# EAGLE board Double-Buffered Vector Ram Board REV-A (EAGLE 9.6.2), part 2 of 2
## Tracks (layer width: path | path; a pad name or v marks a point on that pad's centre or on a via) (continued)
VRAM_B_3 (continued)
  Top 0.508: 6E.13 212.81,13.34 214.08,12.06 216.45,12.06 217.72,13.34 7E.13 238.12,13.34 241.94,17.14 244.39,17.14 245.66,18.41 8E.12 9E.9
VRAM_B_4
  Top 0.508: 6E.14 208.88,15.88 210.15,14.61 216.45,14.61 217.72,15.88 7E.14 238.12,15.88 241.94,19.68 244.39,19.68 245.66,20.95 8E.13 9E.8
VRAM_B_5
  Top 0.508: 6E.15 208.88,18.41 210.15,17.14 216.45,17.14 217.72,18.41 7E.15 235.59,18.41 241.94,24.77 244.39,24.77 245.66,26.04 8E.15 9E.6
VRAM_B_6
  Top 0.508: 6E.16 208.88,20.95 210.15,19.68 216.45,19.68 217.72,20.95 7E.16 233.04,20.95 241.94,29.84 244.39,29.84 245.66,31.11 8E.17 9E.4
VRAM_B_7
  Top 0.508: 6E.17 208.88,23.5 210.15,22.23 216.45,22.23 217.72,23.5 7E.17 241.94,34.92 244.39,34.92 245.66,36.2 8E.19 9E.2
VRAM_B_8
  Top 0.508: 6C.9 205.19,61.59 206.46,62.87 208.83,62.87 210.1,61.59 7C.9 215.67,62 216.81,62 217.67,62.87 231.78,62.87 241.94,73.03 244.47,73.03 245.75,74.3 8C.18 9C.3
VRAM_B_9
  Top 0.508: 6C.10 205.19,59.05 206.46,60.33 208.83,60.33 210.1,59.05 7C.10 215.67,59.46 216.81,59.46 217.67,60.33 234.31,60.33 241.94,67.94 244.39,67.94 245.66,69.22 8C.16 9C.5
VRAM_B_10
  Top 0.508: 6C.11 205.19,56.52 206.46,57.78 208.83,57.78 210.1,56.52 7C.11 215.67,56.92 216.81,56.92 217.67,57.78 236.85,57.78 241.94,62.87 244.47,62.87 245.75,64.14 8C.14 9C.7
VRAM_B_11
  Top 0.381: 6C.13 207.72,53.77 208.83,52.67 229.08,52.67 230.19,53.77 7C.13
  Top 0.508: 7C.13 238.12,53.98 241.94,57.78 244.39,57.78 245.66,59.05 8C.12 9C.9
VRAM_B_12
  Top 0.508: 6C.14 208.88,56.52 210.15,55.24 216.45,55.24 217.72,56.52 7C.14 238.21,56.52 242.02,60.33 244.47,60.33 245.75,61.59 8C.13 9C.8
VRAM_B_13
  Top 0.508: 6C.15 208.88,59.05 210.15,57.78 216.45,57.78 217.72,59.05 7C.15 235.67,59.05 242.02,65.41 244.47,65.41 245.75,66.67 8C.15 9C.6
VRAM_B_14
  Top 0.508: 6C.16 208.88,61.59 210.15,60.33 216.45,60.33 217.72,61.59 7C.16 233.04,61.59 241.94,70.48 244.47,70.48 245.75,71.75 8C.17 9C.4
VRAM_B_15
  Top 0.508: 6C.17 208.88,64.14 210.15,62.87 216.45,62.87 217.72,64.14 7C.17 241.94,75.56 244.47,75.56 245.75,76.83 8C.19 9C.2
VRAMA0  (via drill 0.35)
  Top 0.381: v165.74,100.91 162.05,100.91 4B.11 161.68,101.28 v156.53,101.28 | v156.53,117.49 147.32,117.49 146.95,117.86 124.12,117.86 B1.49
  Bottom 0.381: v165.74,100.91 165.74,22.1 162.05,18.41 4E.11 | v156.53,101.28 v156.53,117.49
VRAMA1  (via drill 0.35)
  Top 0.381: v149.16,27.25 160.58,27.25 161.68,26.15 4E.14 | 4B.14 161.68,108.65 158,112.33 v148.79,112.33 145.11,108.65 119.7,108.65 119.7,116.38 121.17,117.86 B1.48
  Bottom 0.381: v149.16,27.25 149.16,73.29 148.43,74.03 148.43,111.96 v148.79,112.33
VRAMA2  (via drill 0.35)
  Top 0.381: v130.01,51.56 v175.31,51.56 | v130.01,120.43 124.12,120.43 B1.47 | v130.01,116.75 146.22,116.75 146.58,116.38 169.42,116.38 172,113.81 5B.5
  Bottom 0.381: v175.31,51.56 175.31,34.25 172.36,31.3 5E.5 | v130.01,120.43 v130.01,116.75 v130.01,51.56
VRAMA3  (via drill 0.35)
  Top 0.381: v183.78,42.72 176.05,42.72 172.36,39.04 5E.2 | v183.78,125.22 176.05,125.22 172.36,121.54 5B.2 172,121.54 v129.64,121.54 | v90.23,120.8 121.17,120.8 B1.46 | v129.27,160.21 v93.18,160.21
  Bottom 0.381: v183.78,125.22 v183.78,42.72 | v90.23,120.8 90.23,149.53 93.18,152.48 v93.18,160.21 | v129.27,160.21 129.27,125.22 129.64,124.85 v129.64,121.54
VRAMA4  (via drill 0.35)
  Top 0.381: v141.43,61.51 153.95,61.51 4C.5 | v141.8,123.01 124.12,123.01 B1.45
  Bottom 0.381: v141.43,61.51 141.43,122.64 v141.8,123.01 141.8,140.32 152.84,140.32 153.95,141.43 4A.5
VRAMA5  (via drill 0.35)
  Top 0.381: 5C.11 173.1,62.61 v167.94,62.61 | v174.57,103.49 v167.94,103.49 | v175.68,149.9 176.05,150.27 179.36,150.27 5A.11 | v97.6,123.01 121.17,123.01 B1.44 | v89.86,97.6 90.23,97.97 127.8,97.97 130.38,95.39 130.38,90.23 167.58,90.23 v167.94,89.86
  Bottom 0.381: v167.94,103.49 v167.94,89.86 v167.94,62.61 | v174.57,103.49 174.94,103.86 174.94,149.16 v175.68,149.9 | v97.6,123.01 97.6,104.97 90.23,97.6 v89.86,97.6
VRAMA6  (via drill 0.35)
  Top 0.381: v122.28,84.34 v177.52,84.34 | v166.84,154.32 175.68,154.32 179.36,158 5A.14 | v166.84,125.96 124.12,125.96 B1.43
  Bottom 0.381: v177.52,84.34 177.52,78.82 179.36,76.97 5C.14 | v122.28,84.34 122.28,88.76 126.33,92.81 126.33,103.86 126.69,104.23 126.69,123.01 124.12,125.59 B1.43 | v166.84,125.96 v166.84,154.32
VRAMA7  (via drill 0.35)
  Top 0.381: v184.89,80.66 173.47,80.66 172.36,79.55 5C.2 | v184.89,164.63 176.42,164.63 172.73,160.95 172.36,160.95 5A.2 | v71.82,125.96 121.17,125.96 B1.42 | v168.31,163.16 v71.45,163.16
  Bottom 0.381: v184.89,164.63 v184.89,80.66 | v71.82,125.96 71.82,152.48 71.45,152.84 v71.45,163.16 | v168.31,163.16 170.52,160.95 172,160.95 5A.2
VRAMA8  (via drill 0.35)
  Top 0.381: v144.74,75.5 168.31,75.5 172,71.82 5C.5 | v144.74,112.7 124.12,112.7 B1.53 | v144.74,139.22 151,145.48 156.53,145.48 156.53,148.79 162.05,154.32 163.16,154.32 164.26,153.21 172,153.21 5A.5
  Bottom 0.381: v144.74,75.5 v144.74,112.7 v144.74,139.22
VRAMA9  (via drill 0.35)
  Top 0.381: v150.27,73.29 155.42,73.29 161.68,67.03 4C.14 | v149.53,139.22 150.63,140.32 157.26,140.32 159.84,142.9 159.84,146.58 161.68,146.58 4A.14 | v114.54,151.74 114.17,152.11 95.02,152.11 94.28,152.84 94.28,156.53 155.79,156.53 156.16,156.16 v159.84,156.16
  Bottom 0.381: v150.27,73.29 149.16,74.4 149.16,111.23 149.9,111.96 149.9,136.27 149.53,136.64 v149.53,139.22 | v114.54,151.74 114.54,119.7 121.17,113.07 B1.52 | v159.84,156.16 159.84,148.79 161.68,146.95 4A.14
VRAMA10  (via drill 0.35)
  Top 0.381: v188.57,29.83 180.84,29.83 179.73,28.73 5E.11 | v188.57,112.33 188.2,111.96 180.47,111.96 | 180.47,111.96 179.73,111.23 5B.11 | B1.51 124.85,114.54 152.48,114.54 152.84,114.91 164.63,114.91 v165.74,113.81 | v167.94,114.54 170.16,112.33 180.1,112.33 180.47,111.96
  Bottom 0.381: v188.57,112.33 v188.57,29.83 | v165.74,113.81 166.47,114.54 v167.94,114.54
VRAMBANKSELECT  (via drill 0.35)
  Top 0.381: v154.32,123.75 172,123.75 5B.1 | 4A.1 154.32,152.11 154.69,152.48 159.11,152.48 169.79,163.16 172,163.16 5A.1 | v246.39,136.27 265.54,136.27 267.02,137.74 9A.11 | v172.36,168.68 214.35,168.68 v214.72,169.05 | v214.72,164.63 239.4,164.63 243.08,160.95 8A.1 | v261.86,57.82 252.29,57.82 251.18,56.72 8C.11 | v104.97,50.09 99.81,50.09 2D.3 | v104.97,10.68 105.33,11.05 246.02,11.05 250.81,15.84 8E.11 | 9E.1 258.18,37.2 v253.02,37.2 | v260.02,87.66 263.7,87.66 263.7,95.02 267.02,98.34 9B.11
  Bottom 0.381: v154.32,123.75 154.32,113.81 4B.1 | 5B.1 172,124.12 172,142.9 174.21,145.11 174.21,161.31 172.36,163.16 5A.1 172.36,163.53 v172.36,168.68 | 9B.11 267.02,98.7 265.18,100.55 265.18,135.9 267.02,137.74 9A.11 | 8B.1 243.45,121.54 245.66,123.75 245.66,132.59 246.39,133.32 v246.39,136.27 246.39,157.63 243.45,160.58 8A.1 | v214.72,164.63 v214.72,169.05 | 9E.1 261.86,40.88 v261.86,57.82 261.86,77.34 260.02,79.18 9C.1 260.02,79.55 v260.02,87.66 | v104.97,10.68 v104.97,50.09 | v253.02,37.2 253.02,18.05 251.18,16.2 8E.11
VRAMIN0  (via drill 0.35)
  Top 0.381: v262.97,34.99 245.66,34.99 244.55,33.88 243.45,33.88 8E.3 | v262.6,90.6 261.86,91.34 v261.86,92.81 138.48,92.81 138.48,98.7 v139.22,99.44 | v261.86,117.49 245.66,117.49 244.55,116.38 243.45,116.38 8B.3 | v139.22,133.32 124.12,133.32 B1.37
  Bottom 0.381: v262.97,34.99 262.97,90.23 v262.6,90.6 | v261.86,117.49 v261.86,92.81 | v139.22,99.44 v139.22,133.32
VRAMIN1  (via drill 0.35)
  Top 0.381: v254.86,29.83 245.66,29.83 244.55,28.73 243.45,28.73 8E.5 | v254.86,112.33 245.66,112.33 244.55,111.23 243.45,111.23 8B.5 | v118.96,149.53 117.86,150.63 95.39,150.63 93.55,152.48 93.55,157.26 v156.53,157.26 | v156.53,144 157.63,142.9 v158.37,142.9 | v158.74,131.85 185.62,131.85 187.47,133.69 212.88,133.69 214.72,131.85 227.98,131.85 228.35,132.22 244.18,132.22 244.92,131.48 v254.86,131.48
  Bottom 0.381: v254.86,29.83 v254.86,112.33 254.5,112.7 254.5,131.12 v254.86,131.48 | v118.96,149.53 118.59,149.16 118.59,133.32 121.17,133.32 B1.36 | v156.53,144 v156.53,157.26 | v158.37,142.9 158.74,142.53 v158.74,131.85
VRAMIN2  (via drill 0.35)
  Top 0.381: v246.02,46.77 178.26,46.77 177.89,47.14 v140.69,47.14 | B1.35 124.12,135.53 v140.69,135.53 145.48,130.75 185.99,130.75 v186.36,131.12 | v247.5,107.17 245.66,107.17 244.92,106.44 243.81,106.44 243.45,106.07 8B.7 | v186.36,127.06 v247.87,127.06
  Bottom 0.381: v246.02,46.77 246.02,26.15 243.45,23.57 8E.7 | v140.69,47.14 140.32,47.51 140.32,97.6 140.69,97.97 v140.69,135.53 | v247.5,107.17 247.87,107.54 v247.87,127.06 | v186.36,131.12 v186.36,127.06
VRAMIN3  (via drill 0.35)
  Top 0.381: v235.34,14.73 238.29,14.73 241.6,18.05 242.71,18.05 243.08,18.41 8E.9 | v235.34,97.23 235.71,97.6 238.66,97.6 241.97,100.91 243.08,100.91 8B.9 | v76.97,135.53 121.17,135.53 B1.34 | v128.91,98.7 v79.18,98.7 | v130.01,42.35 170.52,42.35 171.63,43.46 183.04,43.46 184.89,45.3 v235.34,45.3
  Bottom 0.381: v235.34,14.73 v235.34,45.3 235.34,76.24 235.71,76.61 235.71,84.34 234.97,85.08 234.97,96.86 v235.34,97.23 | v76.97,135.53 76.61,135.17 76.61,102.76 79.18,100.18 v79.18,98.7 | v128.91,98.7 128.91,46.04 130.01,44.93 v130.01,42.35
VRAMIN4  (via drill 0.35)
  Top 0.381: v238.29,47.88 v247.13,47.88 | v245.66,89.86 246.76,89.86 246.76,86.18 245.66,85.08 238.66,85.08 v238.29,84.71 206.62,84.71 205.14,83.24 v132.59,83.24 | v132.59,137.38 124.85,137.38 124.12,138.11 B1.33
  Bottom 0.381: v247.13,47.88 247.13,24.68 243.45,20.99 8E.8 | v238.29,47.88 238.66,48.25 238.66,84.34 v238.29,84.71 | v245.66,89.86 245.29,90.23 245.29,101.65 243.45,103.49 8B.8 | v132.59,83.24 v132.59,137.38
VRAMIN5  (via drill 0.35)
  Top 0.381: v248.6,27.25 245.66,27.25 244.55,26.15 243.45,26.15 8E.6 | v246.39,99.81 v247.87,98.34 | v50.09,141.43 118.22,141.43 121.17,138.48 B1.32 | v47.51,14.36 47.88,13.99 88.02,13.99 94.28,7.73 v248.6,7.73
  Bottom 0.381: v247.87,98.34 247.5,97.97 247.5,86.18 248.23,85.45 248.23,79.18 247.5,78.45 247.5,64.82 248.97,63.35 248.97,62.24 248.6,61.87 248.6,56.35 248.97,55.98 248.97,50.09 248.6,49.72 v248.6,27.25 v248.6,7.73 | v246.39,99.81 246.02,100.18 246.02,105.7 243.45,108.28 8B.6 | v50.09,141.43 50.09,95.02 47.14,92.08 47.14,64.08 47.51,63.72 v47.51,14.36
VRAMIN6  (via drill 0.35)
  Top 0.381: v236.45,45.67 v244.92,45.67 | v245.29,120.07 v236.08,120.07 | v126.33,130.01 186.73,130.01 189.31,132.59 v208.83,132.59 | v208.83,130.38 209.19,130.01 235.34,130.01 v235.71,130.38
  Bottom 0.381: v244.92,45.67 245.29,45.3 245.29,33.15 243.45,31.3 8E.4 | v236.45,45.67 236.45,84.71 235.71,85.45 235.71,96.13 236.45,96.86 236.45,119.7 v236.08,120.07 235.71,120.43 v235.71,130.38 | v245.29,120.07 245.29,115.65 243.45,113.81 8B.4 | v126.33,130.01 126.33,138.48 124.12,140.69 B1.31 | v208.83,130.38 v208.83,132.59
VRAMIN7  (via drill 0.35)
  Top 0.381: v187.47,39.78 191.15,43.46 236.08,43.46 243.08,36.46 8E.2 | v188.57,130.38 189.67,131.48 213.98,131.48 214.35,131.12 v228.71,131.12 | v228.35,120.07 234.61,120.07 235.71,118.96 243.08,118.96 8B.2 | v89.13,145.11 117.12,145.11 121.17,141.06 B1.30 | v174.57,166.47 v92.08,166.47 | v188.57,169.79 v178.26,169.79
  Bottom 0.381: v187.47,39.78 187.47,129.27 v188.57,130.38 v188.57,169.79 | v228.71,131.12 228.35,130.75 v228.35,120.07 | v89.13,145.11 89.5,145.48 89.5,149.9 92.44,152.84 92.44,159.47 92.08,159.84 v92.08,166.47 | v174.57,166.47 175.68,167.58 175.68,170.16 176.42,170.89 178.26,170.89 v178.26,169.79
VRAMIN8  (via drill 0.35)
  Top 0.381: 264.44,86.55 264.44,87.66 269.23,87.66 274.01,92.44 v274.38,92.44 | 264.44,86.55 264.44,79.18 260.76,75.5 245.66,75.5 244.92,74.77 243.81,74.77 243.45,74.4 8C.3 | v281.38,156.9 245.66,156.9 244.55,155.79 243.45,155.79 8A.3 | v70.71,133.32 v117.49,133.32 | v70.34,159.11 132.22,159.11 132.59,159.47 v134.06,159.47 | v150.63,137.01 v134.06,137.01 | v150.27,93.92 150.63,93.55 248.23,93.55 v248.6,93.92 | 264.44,86.55 v248.6,86.55
  Bottom 0.381: v274.38,92.44 278.44,88.39 281.75,88.39 281.75,112.7 281.38,113.07 v281.38,156.9 | v117.49,133.32 117.49,149.53 118.59,150.63 118.59,151 121.17,151 B1.22 | v70.71,133.32 70.71,158.74 v70.34,159.11 | v134.06,137.01 v134.06,159.47 | v150.63,137.01 150.63,94.28 v150.27,93.92 | v248.6,93.92 248.23,93.55 248.23,86.92 v248.6,86.55
VRAMIN9  (via drill 0.35)
  Top 0.381: v245.66,88.02 245.66,87.66 246.02,87.29 246.02,86.55 245.29,85.81 v236.82,85.81 | v128.54,124.48 128.91,124.85 170.52,124.85 174.94,129.27 v236.82,129.27
  Bottom 0.381: v245.66,88.02 246.02,87.66 246.02,71.82 243.45,69.24 8C.5 | v236.82,85.81 236.45,86.18 236.45,95.76 237.19,96.5 237.19,129.27 | 237.19,129.27 237.19,135.53 236.45,136.27 236.45,167.94 238.66,170.16 241.24,170.16 241.24,157.63 241.97,156.9 245.29,156.9 245.29,152.48 243.45,150.63 8A.5 | v128.54,124.48 128.54,146.58 124.12,151 B1.23 | 237.19,129.27 v236.82,129.27
VRAMIN10  (via drill 0.35)
  Top 0.381: v248.6,65.19 245.66,65.19 244.92,64.45 243.45,64.45 8C.7 | v261.86,78.82 261.12,78.08 v248.6,78.08 v228.35,78.08 | v248.97,125.96 v262.6,125.96 | v248.6,146.58 248.23,146.22 245.29,146.22 244.55,145.48 243.45,145.48 8A.7 | v113.44,148.79 113.81,148.43 121.17,148.43 B1.24 | v113.44,107.17 119.33,107.17 120.8,105.7 120.8,102.39 143.27,102.39 v143.64,102.76 | v228.35,86.55 v143.64,86.55
  Bottom 0.381: v248.6,78.08 v248.6,65.19 | v261.86,78.82 262.23,79.18 262.23,89.5 261.49,90.23 261.49,90.97 262.97,92.44 262.97,125.59 v262.6,125.96 | v248.97,125.96 248.97,137.01 248.6,137.38 v248.6,146.58 | v113.44,107.17 v113.44,148.79 | v143.64,86.55 v143.64,102.76 | v228.35,78.08 v228.35,86.55
VRAMIN11  (via drill 0.35)
  Top 0.381: v237.55,52.67 v244.92,52.67 | v237.55,83.6 245.29,83.6 247.5,85.81 247.5,90.97 v237.55,90.97 237.19,91.34 208.46,91.34 207.72,90.6 206.99,90.6 206.62,90.97 131.85,90.97 v131.48,91.34 | v237.55,136.64 238.29,136.64 241.97,140.32 243.08,140.32 8A.9 | v131.48,148.43 124.12,148.43 B1.25
  Bottom 0.381: v244.92,52.67 245.29,53.03 245.29,57.09 243.45,58.93 8C.9 | v237.55,83.6 v237.55,52.67 | v237.55,90.97 237.92,91.34 237.92,136.27 v237.55,136.64 | v131.48,91.34 v131.48,148.43
VRAMIN12  (via drill 0.35)
  Top 0.381: v245.66,49.35 v227.98,49.35 v135.9,49.35 | v245.29,133.69 v227.24,133.69 | v61.14,134.43 v119.7,134.43 | v61.14,107.17 59.66,107.17 58.56,106.07 58.56,103.86 v69.61,103.86 | v135.9,62.24 v69.61,62.24
  Bottom 0.381: v245.66,49.35 246.02,49.72 246.02,58.93 243.45,61.51 8C.8 | v227.98,49.35 227.98,76.97 223.19,81.76 223.19,103.12 227.24,107.17 v227.24,133.69 | v245.29,133.69 245.29,140.69 243.45,142.53 8A.8 | v119.7,134.43 119.7,144.37 121.17,145.85 B1.26 | v61.14,107.17 v61.14,134.43 | v69.61,62.24 v69.61,103.86 | v135.9,49.35 v135.9,62.24
VRAMIN13  (via drill 0.35)
  Top 0.381: v247.87,62.61 v245.66,62.61 | v218.03,50.46 v247.87,50.46 | v246.76,125.96 v217.3,125.96 | v247.5,149.16 247.13,148.79 245.29,148.79 244.55,148.06 243.45,148.06 8A.6 | v130.38,146.22 124.12,146.22 B1.27 | v130.38,168.68 94.28,168.68 93.55,169.42 93.55,170.89 247.13,170.89 v247.5,170.52
  Bottom 0.381: v245.66,62.61 245.66,64.45 243.45,66.66 8C.6 | v247.87,50.46 v247.87,62.61 | v218.03,50.46 218.03,84.71 221.72,88.39 221.72,110.12 217.3,114.54 v217.3,125.96 | v246.76,125.96 246.76,132.59 247.5,133.32 v247.5,149.16 v247.5,170.52 | v130.38,168.68 v130.38,146.22
VRAMIN14  (via drill 0.35)
  Top 0.381: v244.92,86.92 v238.29,86.92 234.97,90.23 v208.83,90.23 | v132.96,158.37 92.81,158.37 92.81,152.11 97.23,147.69 117.12,147.69 121.17,143.64 B1.28 | v134.8,92.08 135.17,91.71 v207.35,91.71
  Bottom 0.381: v244.92,86.92 245.29,86.55 245.29,73.66 243.45,71.82 8C.4 | v238.29,86.92 238.66,87.29 238.66,167.58 238.29,167.94 238.29,168.68 239.03,169.42 240.5,169.42 240.5,155.79 243.08,153.21 8A.4 | v132.96,158.37 132.96,159.84 133.69,160.58 135.17,160.58 135.17,99.81 134.8,99.44 v134.8,92.08 | v208.83,90.23 v207.35,91.71
VRAMIN15  (via drill 0.35)
  Top 0.381: v234.61,76.97 243.08,76.97 8C.2 | v234.61,158 243.08,158 8A.2 243.45,158.37 244.18,159.11 245.29,159.11 245.29,160.95 240.5,165.74 186.36,165.74 v185.99,165.37 | v185.99,133.69 184.89,132.59 160.95,132.59 160.58,132.96 158.37,132.96 156.9,131.48 146.22,131.48 145.85,131.85 145.48,131.85 145.48,132.96 146.22,133.69 151.74,133.69 151.74,137.38 151,138.11 144.37,138.11 144,138.48 128.91,138.48 124.12,143.27 B1.29
  Bottom 0.381: v234.61,76.97 234.24,77.34 234.24,157.63 v234.61,158 | v185.99,165.37 v185.99,133.69
VRAMPC  (via drill 0.35)
  Top 0.381: v122.28,28.73 117.49,28.73 3E.2 | v122.28,53.77 117.49,53.77 3D.2 | v122.28,79.18 117.49,79.18 3C.2 117.12,79.55 v113.44,79.55 | v280.28,118.96 296.11,118.96 P1.D | v280.28,169.42 216.56,169.42 215.09,167.94 173.1,167.94 172.73,167.58 v135.9,167.58 | v135.9,99.07 135.17,99.81 v113.44,99.81
  Bottom 0.381: v122.28,28.73 v122.28,53.77 v122.28,79.18 | v280.28,169.42 v280.28,118.96 | v135.9,99.07 v135.9,167.58 | v113.44,79.55 v113.44,99.81
WE_A  (via drill 0.35)
  Top 0.508: 7B.21 217.72,116.2 216.45,114.94 210.15,114.94 208.88,116.2 6B.21 207.24,115.8 206.1,115.8 205.24,114.94 v202.56,114.94 | 7A.21 217.72,155.57 216.45,154.31 210.15,154.31 208.88,155.57 6A.21 207.24,155.17 206.1,155.17 205.24,154.31 v202.56,154.31 191.22,154.31 188.04,151.12 188.04,146.31 175.71,133.99 4A.9
  Bottom 0.508: v202.56,114.94 v202.56,154.31
WE_B  (via drill 0.35)
  Top 0.508: 7C.21 217.72,74.3 216.45,73.03 210.15,73.03 208.88,74.3 6C.21 207.24,73.89 206.1,73.89 205.24,73.03 v202.56,73.03 191.22,73.03 188.59,70.4 188.59,65.59 176.98,53.98 4C.9 | 7E.21 217.72,33.66 216.45,32.38 210.15,32.38 208.88,33.66 6E.21 207.24,33.25 206.1,33.25 205.24,32.38 v202.56,32.38
  Bottom 0.508: v202.56,32.38 v202.56,73.03
WEIN  (via drill 0.35)
  Top 0.381: v175.31,59.3 162.05,59.3 4C.11 | v176.05,138.85 162.05,138.85 4A.11 | v96.5,128.54 121.17,128.54 B1.40 | v176.78,169.79 v94.65,169.79
  Bottom 0.381: v175.31,59.3 175.68,59.66 175.68,138.48 v176.05,138.85 176.78,139.59 v176.78,169.79 | v96.5,128.54 96.5,141.8 94.28,144 94.28,169.42 v94.65,169.79

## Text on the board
Top: Double-Buffered Vector RAM Board | (C) Kincaid Arcade 6/8/2020 | KincaidArcade.com | Designed By: Alexander K. Haley | (A 17 year old!) | Board and design licensed under CC BY-SA 4.0 | https://creativecommons.org/licenses/by-sa/4.0/
tPlace: A | B | C | D | E | 1 | 2 | 3 | 4 | 5 | 6 | 7 | 8 | 9
bPlace: A | B | C | D | E | 1 | 2 | 3 | 4 | 5 | 6 | 7 | 8 | 9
